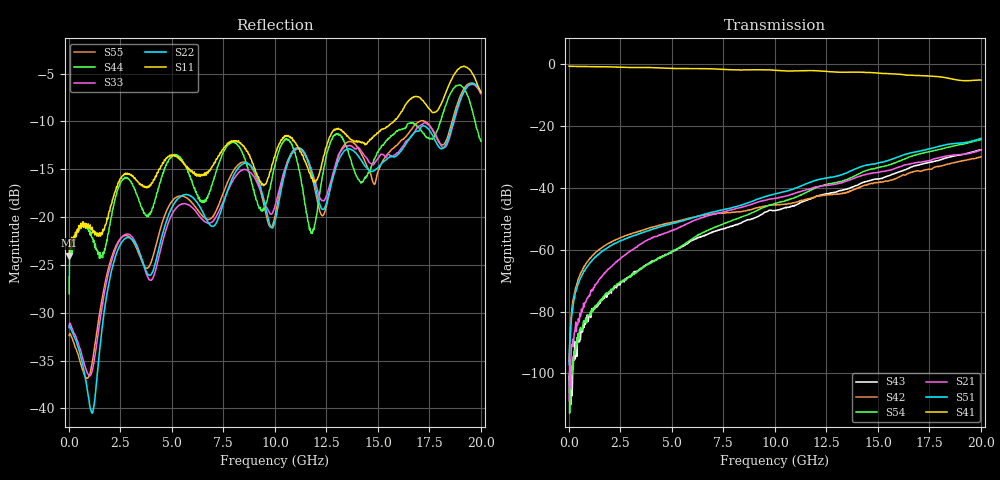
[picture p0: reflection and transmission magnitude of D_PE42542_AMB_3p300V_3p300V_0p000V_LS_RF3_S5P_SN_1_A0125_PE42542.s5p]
! Device ID: PE42542
! Device ID: PE42542
! File Path: z:\PE42542\PE42543_20140723_inv\AMB\3p300\LS_RF3\PE42542_AMB_3p300V_3p300V_0p000V_LS_RF3_S5P_SN_1_A0125_PE42542.s5p
! Serial: 1
! Lot: A0125_PE42542
! Temp: AMB
! VDD: 3.300
! VSS: 0.000
! Control_Hi: 3.300
! Control_Lo: 0.000
! Logic State: LS_RF3
! Port 1: RFC
! Port 2: RF1
! Port 3: RF2
! Port 5: RF3
! Port 6: RF4
! ThroughPath:1-5
! IDD: -0.000143372956
! ISS: 4.23013998e-012
#  Hz  S  RI  R  50
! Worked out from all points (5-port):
!   801 points, 10 MHz to 20 GHz, reference 50 ohm
!   strongest paths, dB at 10 MHz, 5.008 GHz, 10.01 GHz, 15 GHz, 20 GHz:
!     S41: -0.6, -1.4, -2.0, -2.9, -5.1
!     S51: -97.1, -51.5, -41.9, -31.9, -24.0
!     S21: -108.8, -53.7, -43.4, -35.0, -27.8
!     S54: -100.1, -60.7, -45.1, -33.4, -24.4
!     S42: -96.2, -51.1, -45.5, -38.3, -29.9
!     S43: -100.9, -60.6, -47.3, -37.1, -27.7
!   lowest |S11| = -24.0 dB at 10 MHz (marker M1), VSWR 1.13, Z = 56.1 - j2.8 ohm
!   |S11| at or under -10 dB: start of sweep to 15.77 GHz
